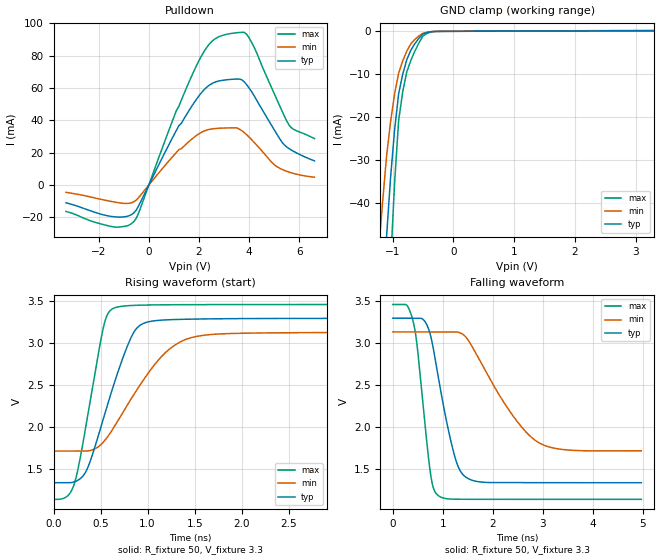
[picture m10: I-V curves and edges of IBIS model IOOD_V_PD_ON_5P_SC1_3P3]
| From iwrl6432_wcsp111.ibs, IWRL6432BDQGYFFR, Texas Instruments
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|   Model Cell IOOD_V_PD_ON_5P_SC1_3P3
|IOOD_V_PD_ON_5P_SC1_3P3
[Model]   IOOD_V_PD_ON_5P_SC1_3P3
Model_type   I/O_open_drain
Polarity   Non-Inverting
Enable   Active-Low
Vinl =  0.8V
Vinh =  2V
Cref =  15pF
Rref =  100.0000M
Vref =  0V
Vmeas =  1.65
|   typ   min   max
C_comp   2.059994p   1.862014p   2.067327p
[Model Spec]
Vinl   0.8V   0.8V   0.8V
Vinh   2V   2V   2V
[Temperature Range]   25   125   -40
[Voltage Range]   3.3   3.135   3.465
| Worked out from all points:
|   slope of the pulldown table from 0 to 0.495 V, typ, clamps not added: 31.8 ohm
|   GND clamp passes 1 mA (typ) near -0.52 V on its own axis
|   rising waveform, R_fixture 50, V_fixture 3.3: 20-80 % time 334ps typ, 511ps min, 217ps max; typ from 1.33 V to 3.3 V
|   falling waveform, R_fixture 50, V_fixture 3.3: 20-80 % time 385ps typ, 889ps min, 239ps max; typ from 3.3 V to 1.33 V
| Where Nom  PVT is Nominal Process, 3.3V, 25C
|   Fast PVT is Strong Process,  3.465V, -40C
|   Slow PVT is Weak Process,   3.135V, 125C
[Pulldown]
|   voltage   I(typ)   I(min)   I(max)
-3.3V     -10.93mA   -4.474mA   -16.27mA
-1.4V     -19.53mA   -10.38mA   -25.83mA
-600mV    -17.23mA   -10.34mA   -22.61mA
1.2V      36.72mA    21.93mA    48.76mA
1.9V      53.02mA    30.66mA    73.76mA
2.4V      61.61mA    34.34mA    86.89mA
3V        64.86mA    35.24mA    92.76mA
3.6V      65.51mA    34.65mA    94.24mA
3.9V      62.01mA    31.1mA     93.16mA
5V        34.1mA     12.57mA    56.42mA
5.6V      22.42mA    7.958mA    36.79mA
6.6V      14.97mA    4.886mA    28.74mA
[GND_clamp]
|   voltage   I(typ)   I(min)   I(max)
-3.3V     -787.2mA   -627.7mA   -1.235A
-1.233V   -85.66mA   -52.14mA   -138.8mA
-1.167V   -66.47mA   -40.37mA   -107.7mA
-1.1V     -48.25mA   -29.37mA   -77.98mA
-1.033V   -34.28mA   -21.19mA   -54.56mA
-966.7mV  -23.07mA   -14.67mA   -35.51mA
-900mV    -14.62mA   -9.792mA   -20.84mA
-833.3mV  -10.07mA   -6.939mA   -14.17mA
-700mV    -4.435mA   -2.94mA    -6.836mA
-500mV    -641.2uA   -454.9uA   -1.12mA
-300mV    -31.62uA   -32.88uA   -44.11uA
3.3V      108.6uA    60.68uA    188uA
[Ramp]
| variable   typ   min   max
dV/dt_f  1.1800539/0.38506826n 0.85624661/0.8953951n  1.3975801/0.23949187n
dV/dt_r  1.1731735/0.46682557n   0.861622/1.0170237n   1.40552/0.25245197n
R_load = 50
[Rising Waveform]
R_fixture = 50
V_fixture = 3.3
V_fixture_min = 3.135
V_fixture_max = 3.465
|   time   V(typ)   V(min)   V(max)
0s        1.335V     1.713V     1.137V
145.7ps   1.335V     1.713V     1.174V
223.8ps   1.347V     1.713V     1.333V
354.7ps   1.492V     1.713V     2.079V
528.6ps   2.096V     1.819V     3.182V
642.8ps   2.515V     1.999V     3.419V
908.7ps   3.205V     2.483V     3.454V
1.202ns   3.279V     2.902V     3.459V
1.488ns   3.288V     3.073V     3.46V
4.974ns   3.298V     3.131V     3.462V
[Falling Waveform]
R_fixture = 50
V_fixture = 3.3
V_fixture_min = 3.135
V_fixture_max = 3.465
|   time   V(typ)   V(min)   V(max)
0s        3.298V     3.134V     3.461V
276.8ps   3.298V     3.134V     3.454V
412.9ps   3.298V     3.134V     3.243V
749.7ps   3.105V     3.134V     1.462V
910.7ps   2.593V     3.134V     1.18V
1.252ns   1.623V     3.134V     1.138V
1.512ns   1.382V     3.033V     1.136V
2.315ns   1.336V     2.209V     1.136V
2.892ns   1.335V     1.823V     1.136V
4.974ns   1.334V     1.716V     1.136V
